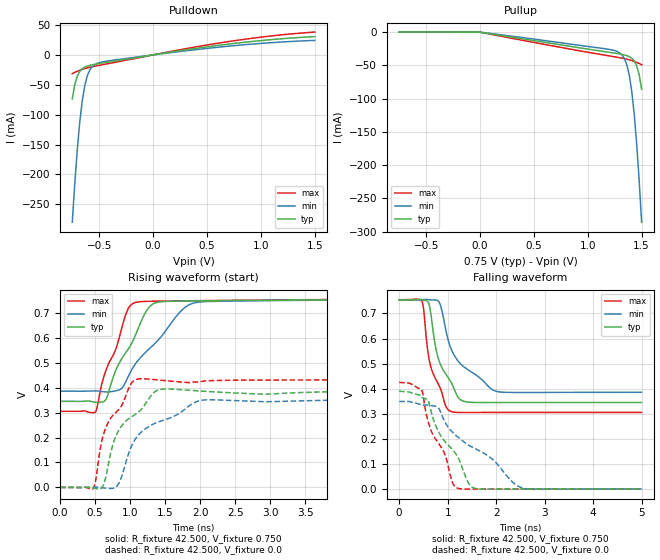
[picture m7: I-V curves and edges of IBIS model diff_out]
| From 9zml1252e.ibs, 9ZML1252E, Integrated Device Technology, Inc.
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|   Model diff_out (clk_out0914_all.ibs)
[Model] diff_out
Model_type Output
Polarity   Non-Inverting
Vmeas =  0.200V
Cref =  0.0F
Rref =  50.000
Vref =  0.350V
C_comp   2.000pF   2.000pF   2.000pF
[Temperature Range]   65.000   0.125k   -10.000
[Voltage Range]   0.750V   0.750V   0.750V
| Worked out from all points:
|   slope of the pulldown table from 0 to 0.112 V, typ, clamps not added: 34.7 ohm
|   slope of the pullup table from 0 to 0.112 V, typ, clamps not added: 41 ohm
|   rising waveform, R_fixture 42.500, V_fixture 0.750: 20-80 % time 427ps typ, 643ps min, 326ps max; typ from 0.345 V to 0.753 V
|   rising waveform, R_fixture 42.500, V_fixture 0.0: 20-80 % time 477ps typ, 696ps min, 370ps max; typ from 0 V to 0.389 V
|   falling waveform, R_fixture 42.500, V_fixture 0.750: 20-80 % time 395ps typ, 634ps min, 331ps max; typ from 0.753 V to 0.345 V
|   falling waveform, R_fixture 42.500, V_fixture 0.0: 20-80 % time 658ps typ, 1.23ns min, 498ps max; typ from 0.39 V to 0 V
[Pulldown]
|Voltage   I(typ)   I(min)   I(max)
-750mV    -73.54mA   -280mA     -31.41mA
-727mV    -49.86mA   -215.7mA   -29.24mA
-704mV    -35.61mA   -159.7mA   -27.36mA
-681mV    -27.57mA   -113.3mA   -25.7mA
-658mV    -23.08mA   -77.62mA   -24.22mA
-635mV    -20.45mA   -52.29mA   -22.91mA
-612mV    -18.77mA   -35.76mA   -21.75mA
-589mV    -17.58mA   -25.68mA   -20.73mA
-543mV    -15.82mA   -16.28mA   -18.94mA
-382mV    -11.06mA   -9.178mA   -13.4mA
630mV     16.48mA    13.32mA    20.34mA
1.5V      30.55mA    24.24mA    38.18mA
[Pullup]
|Voltage   I(typ)   I(min)   I(max)
-750mV    76.75uA    66.9uA     89.69uA
5mV       -156.9uA   -129.2uA   -204uA
1.178V    -29.81mA   -25.42mA   -35.14mA
1.293V    -32.73mA   -30.77mA   -38.34mA
1.339V    -34.25mA   -39.45mA   -39.8mA
1.362V    -35.3mA    -48.85mA   -40.65mA
1.385V    -36.8mA    -64.4mA    -41.62mA
1.408V    -39.15mA   -88.47mA   -42.73mA
1.431V    -43.22mA   -122.8mA   -44.01mA
1.454V    -50.57mA   -167.7mA   -45.46mA
1.477V    -63.73mA   -222.5mA   -47.11mA
1.5V      -85.88mA   -285.8mA   -49.03mA
[Ramp]
| variable   typ   min   max
dV/dt_r   0.233/0.181n   0.211/0.196n   0.256/0.179n
dV/dt_f   0.243/0.395n   0.219/0.621n   0.267/0.320n
R_load = 42.500
[Rising Waveform]
R_fixture= 42.500
V_fixture= 0.750
V_fixture_min= 0.750
V_fixture_max= 0.750
|time   V(typ)   V(min)   V(max)
0s        345mV      385.7mV    305.3mV
510ps     341mV      386.8mV    305.3mV
653ps     352.4mV    382.8mV    468.2mV
856ps     504.2mV    392.3mV    613mV
967ps     551.9mV    441.2mV    713.2mV
1.066ns   604mV      491.4mV    740.2mV
1.313ns   732.9mV    566.1mV    746mV
1.706ns   746.5mV    701.1mV    747.4mV
1.906ns   747.2mV    738.8mV    748.1mV
5ns       753.2mV    752.6mV    754.7mV
[Rising Waveform]
R_fixture= 42.500
V_fixture= 0.0
V_fixture_min= 0.0
V_fixture_max= 0.0
|time   V(typ)   V(min)   V(max)
0s        33.71uV    28.39uV    23.3uV
474ps     -2.001mV   1.23mV     -3.518mV
592ps     -2.067mV   -565.9uV   182.5mV
653ps     43.06mV    -2.86mV    239.6mV
743ps     161.6mV    -3.863mV   285.6mV
814ps     216.6mV    6.396mV    305.2mV
1.094ns   296.5mV    201.8mV    433.2mV
1.383ns   388.5mV    260.3mV    431.1mV
2.024ns   386mV      349.4mV    424.6mV
5ns       389.3mV    353.1mV    431mV
[Falling Waveform]
R_fixture= 42.500
V_fixture= 0.750
V_fixture_min= 0.750
V_fixture_max= 0.750
|time   V(typ)   V(min)   V(max)
0s        753.3mV    752.8mV    754.7mV
470ps     754.2mV    755mV      749mV
510ps     752.7mV    755.6mV    707.5mV
591ps     747.8mV    755.3mV    550.2mV
641ps     713.8mV    754.4mV    496.1mV
805ps     522.4mV    749.7mV    419.3mV
1.06ns    429.2mV    564.6mV    310mV
1.293ns   352.9mV    494.1mV    305.1mV
2.005ns   344.8mV    389.4mV    305.3mV
5ns       345mV      385.7mV    305.3mV
[Falling Waveform]
R_fixture= 42.500
V_fixture= 0.0
V_fixture_min= 0.0
V_fixture_max= 0.0
|time   V(typ)   V(min)   V(max)
0s        389.9mV    349.1mV    425.1mV
470ps     364.1mV    333.7mV    392.1mV
593ps     354mV      334.2mV    272.4mV
660ps     308.5mV    332.6mV    232.6mV
863ps     210.5mV    302.9mV    167.4mV
1.1ns     156.9mV    226.3mV    26.09mV
1.205ns   129mV      208.3mV    3.32mV
1.533ns   4.63mV     164.3mV    -100.7uV
2.555ns   33.56uV    3.522mV    59.13uV
5ns       33.73uV    28.53uV    23.3uV
